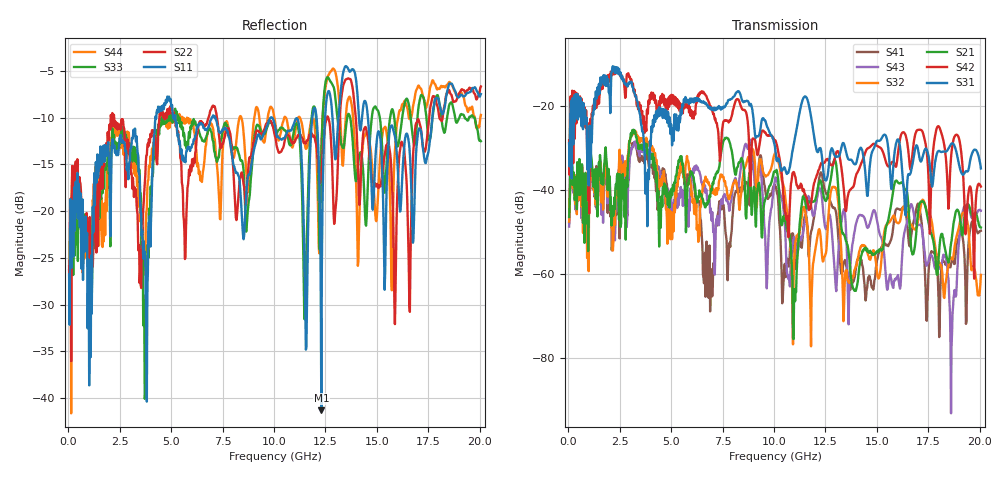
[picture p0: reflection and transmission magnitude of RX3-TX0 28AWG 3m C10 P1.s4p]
! FILE: O:\PROJECTS\SI-2007-05-003 3m Eyemax Qual\XT\FD\RX3-TX0 28AWG 3m C10 P1.s4p
# MHZ S RI R 50.00
! FREQ  S11  S12  S13  S14
!  S21  S22  S23  S24
!  S31  S32  S33  S34
!  S41  S42  S43  S44
!  REAL  IMAG  REAL  IMAG  REAL  IMAG  REAL  IMAG
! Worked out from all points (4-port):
!   801 points, 50 MHz to 20.05 GHz, reference 50 ohm
!   strongest paths, dB at 50 MHz, 5.05 GHz, 10.05 GHz, 15.05 GHz, 20.05 GHz:
!     S31: -28.9, -29.4, -29.8, -28.3, -34.9
!     S42: -28.2, -19.3, -28.4, -29.6, -39.2
!     S21: -46.5, -41.3, -35.7, -54.4, -49.0
!     S32: -47.6, -51.7, -31.3, -60.8, -60.2
!     S43: -48.7, -43.3, -37.8, -48.4, -45.0
!     S41: -47.8, -45.7, -38.9, -55.8, -49.7
!   lowest |S11| = -41.3 dB at 12.3 GHz (marker M1), VSWR 1.02, Z = 50.3 - j0.818 ohm
!   |S11| at or under -10 dB: start of sweep to 4.244 GHz; 7.154 GHz to 9.845 GHz (2.691 GHz wide, 31.7 % of centre); 14.56 GHz to 17.69 GHz (3.125 GHz wide, 19.4 % of centre)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
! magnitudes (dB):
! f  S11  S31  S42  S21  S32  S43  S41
! 50 MHz  -26.8  -28.9  -28.2  -46.5  -47.6  -48.7  -47.8
! 7.7 GHz  -11.4  -19.4  -23.5  -27.6  -39.5  -42.7  -52.1
! 10.1 GHz  -11.5  -32.1  -28.6  -35.8  -31.8  -37.3  -39.3
! 11 GHz  -10.4  -28.2  -36.4  -63.6  -54.8  -52.0  -54.7
! 12.3 GHz  -41.3  -31.0  -33.6  -38.4  -53.5  -40.6  -36.0
! 18.62 GHz  -6.4  -29.0  -31.0  -52.1  -56.4  -77.0  -57.0
! 20.05 GHz  -7.5  -34.9  -39.2  -49.0  -60.2  -45.0  -49.7
